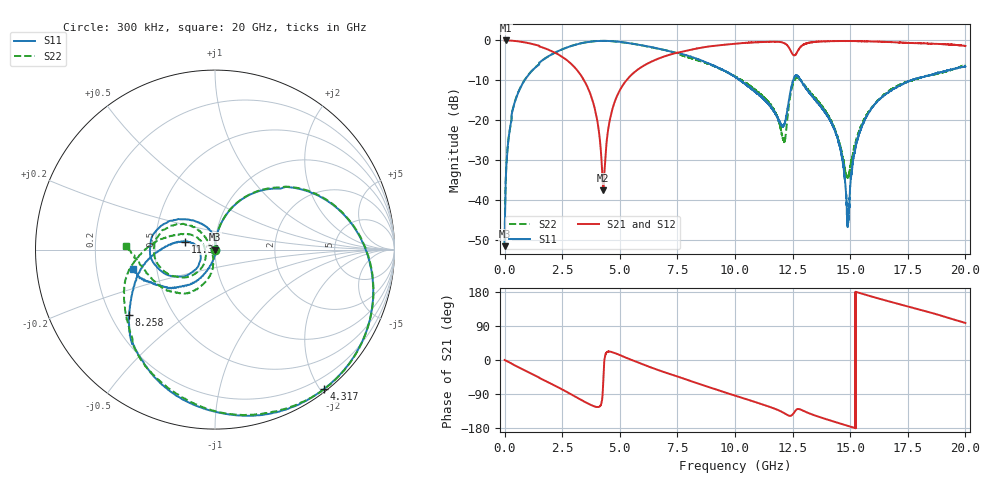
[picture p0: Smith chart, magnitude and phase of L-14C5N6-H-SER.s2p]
!{L-14C5N6}
!Johanson Technology Inc.
!www.johansontechnology.com
!Test Board Conditions:
!Substrate Type  RO4350B
!Substrate Thickness  20 mil
!Substrate Dk  3.66
!TL Type: GCPW
!TL Trace Width  36 mil
!TL Gap  12 mil
!Electrode orientation  Horizontal
!DUT TOPOLOGY	SERIES
!Mounting Pad LxW  26x36 mil
! Created Sun Jun 20 12:58:32 2021
# hz S ma R 50
! 2 Port Network Data from SP1.SP block
! freq  magS11  angS11  magS21  angS21  magS12  angS12  magS22  angS22
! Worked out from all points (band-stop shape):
!   20001 points, 300 kHz to 20 GHz, reference 50 ohm
!   highest |S21| = -0.01 dB at 69.3 MHz (marker M1); lowest = -37.7 dB at 4.284 GHz (marker M2)
!   |S21| within 3 dB of the highest: 7.573 GHz to 12.45 GHz (4.88 GHz wide, 48.7 % of centre); 12.69 GHz to end of sweep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
!   lowest |S11| = -51.6 dB at 1.3 MHz (marker M3), VSWR 1.01, Z = 49.7 + j0.0273 ohm
!   |S11| at or under -10 dB: start of sweep to 868 MHz; 10.22 GHz to 12.52 GHz (2.303 GHz wide, 20.2 % of centre); 12.86 GHz to 17.64 GHz (4.781 GHz wide, 31.4 % of centre)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
!   |S22| runs from -51.5 to -0.1 dB; largest |S21 - S12| = 0.016
!   S11 on the Smith chart (normalised r, x): 300 kHz: 0.99, -0.00; 4.317 GHz: 0.04, -2.05; 8.258 GHz: 0.28, -0.31; 11.36 GHz: 0.71, +0.07; 20 GHz: 0.36, -0.10
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300000  0.002678 -176.2  0.9977 0.0  0.9969 0.0  0.002649 -178.9
1300000  0.00262 174.0  0.9975 -0.0  0.9972 -0.1  0.002733 169.2
6.93e7  0.02426 91.6  0.9985 -2.1  0.9976 -2.2  0.02464 91.4
2.943e8  0.09862 81.6  0.994 -9.0  0.9936 -8.8  0.1001 81.7
7.513e8  0.2772 65.6  0.9569 -23.7  0.9577 -23.7  0.2793 65.8
3.3343e9  0.9233 -17.7  0.3568 -105.6  0.3579 -105.6  0.9226 -17.0
3.9313e9  0.9787 -38.7  0.1329 -123.0  0.1329 -123.1  0.979 -38.1
4.2843e9  0.9859 -50.9  0.01309 -51.1  0.01334 -51.6  0.9876 -50.0
4.3173e9  0.9862 -52.1  0.0177 -9.9  0.01789 -9.7  0.9871 -51.1
4.9353e9  0.9634 -71.9  0.2173 14.6  0.2179 14.9  0.9587 -70.7
6.6673e9  0.791 -114.6  0.5894 -26.6  0.5905 -26.3  0.7856 -114.6
8.2583e9  0.6005 -142.7  0.7817 -59.2  0.7857 -58.9  0.5768 -151.5
1.00003e10  0.3492 -174.5  0.908 -94.1  0.9097 -94.1  0.3542 175.2
1.13573e10  0.171 164.9  0.9577 -120.5  0.9589 -120.7  0.1804 151.0
1.21153e10  0.08519 -158.7  0.9312 -139.5  0.9307 -139.6  0.05438 -176.8
1.26023e10  0.3559 -170.2  0.6518 -135.5  0.6561 -135.7  0.324 -163.9
1.33343e10  0.2019 126.5  0.9482 -143.4  0.9449 -143.4  0.2112 139.1
1.44003e10  0.06491 94.0  0.981 -164.5  0.9808 -164.6  0.06757 128.3
1.49003e10  0.005454 -8.5  0.983 -173.9  0.9828 -173.8  0.01909 -154.5
1.54583e10  0.07557 -103.9  0.9779 176.0  0.9786 175.9  0.08284 -96.6
1.66673e10  0.222 -124.0  0.9549 155.1  0.9488 154.9  0.2315 -113.0
2e10  0.4704 -166.6  0.852 97.7  0.8397 97.4  0.4957 177.4
